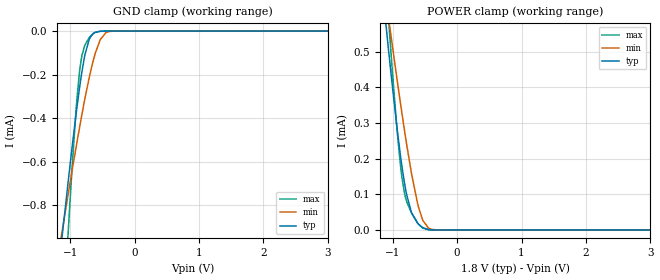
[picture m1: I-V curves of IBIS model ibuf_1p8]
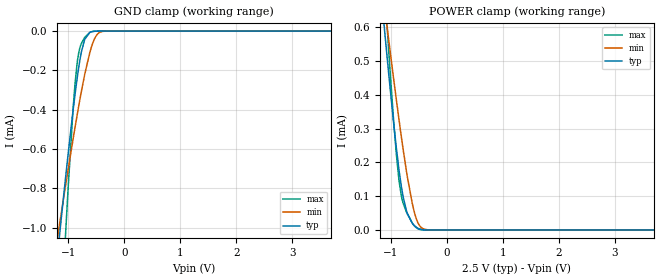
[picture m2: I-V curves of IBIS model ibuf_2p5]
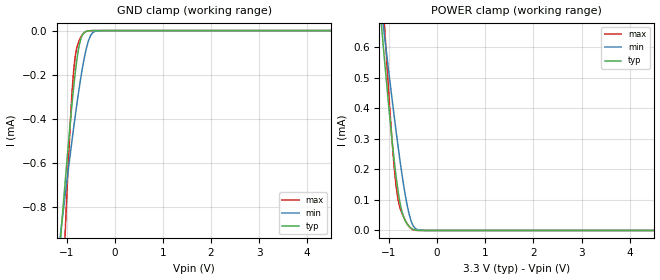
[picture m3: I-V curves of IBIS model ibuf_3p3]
|Texas Instruments Incorporated
|ISO7041 Ultra-Low Power Four-Channel Digital Isolator
[IBIS Ver]   4.1
[File name]   iso7041.ibs
[Date]   12/18/2018
[File Rev]   1.0
[Source]
| Texas Instruments Incorporated.
| Analog-eLab Design Center, HPA
| 12500 TI Blvd
| Dallas, TX -75243
[Notes]   Revision History:
| Rev 1.0: 12/18/2018
| - Initial version of the model
| - Model generated from simulations in SPECTRE
| - Warnings regarding combined Non-monotonicity of various models
|   have been reviewed and considered minor and can be ignored.
| - Model names with a trailing _1p8 contain the model for 1.8V operation.
|   Model names with a trailing _2p5 contain the model for 2.5 operation.
|   Model names with a trailing _3p3 contain the model for 3.3V operation.
|   Model names with a trailing _5p0 contain the model for 5.0V operation.
| - C_comp although listed in numerical order of value are
|   obtained from varying PVT conditions. For PVT conditions for
|   each specific value refer the buffer description under
|   respective [Model]. IBIS model user is responsible for using
|   appropriate C_comp to simulate for Signal Integrity.
[Disclaimer]
| This model is designed as an aid for customers of Texas Instruments.
| TI and its licensors and suppliers make no warranties, either expressed
| or implied, with respect to this  model, including the warranties of
| merchantability or fitness for a particular purpose. The model is
| provided solely on an "as is" basis. The entire risk as to its quality
| and performance is with the customer.
| This model is subject to change without notice. Texas Instruments
| Incorporated is not responsible for updating this model.
[Copyright]
(C) Copyright 2018 Texas Instruments Incorporated.All rights reserved.
|  Component ISO7041DBQ 16-pin QSOP - DBQ package
|  Part # ISO7041DBQ
[Component]   ISO7041DBQ
[Manufacturer]  TI
[Package]   |16 QSOP - DBQ package
|   typ   min   max
R_pkg   0.05   0.04   0.06
L_pkg   1.0nH   0.8nH   1.2nH
C_pkg   0.2pF   0.16pF   0.24pF
[Pin]  signal_name  model_name   R_pin   L_pin   C_pin
1   VCC1   power   NA   NA   NA
2   GND1   gnd   NA   NA   NA
3   INA   ibuf   NA   NA   NA
4   INB   ibuf   NA   NA   NA
5   INC   ibuf   NA   NA   NA
6   OUTD   obuf   NA   NA   NA
7   EN1   ibuf   NA   NA   NA
8   GND1   gnd   NA   NA   NA
9   GND2   gnd   NA   NA   NA
10   EN2   ibuf   NA   NA   NA
11   IND   ibuf   NA   NA   NA
12   OUTC   obuf   NA   NA   NA
13   OUTB   obuf   NA   NA   NA
14   OUTA   obuf   NA   NA   NA
15   GND2   gnd   NA   NA   NA
16   VCC2   power   NA   NA   NA
|   Model Selectors
[Model Selector] ibuf
ibuf_1p8   1.8V   digital Input
ibuf_2p5   2.5V   digital Input
ibuf_3p3   3.3V   digital Input
ibuf_5p0   5.0V   digital Input
[Model Selector] obuf
obuf_1p8   1.8V   digital Output
obuf_2p5   2.5V   digital Output
obuf_3p3   3.3V   digital Output
obuf_5p0   5.0V   digital Output
| Models and submodels in the file (8): ibuf_1p8 (Input), ibuf_2p5 (Input), ibuf_3p3 (Input), ibuf_5p0 (Input), obuf_1p8 (3-state), obuf_2p5 (3-state), obuf_3p3 (3-state), obuf_5p0 (3-state)
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|   ibuf_1p8 Model
[Model]   ibuf_1p8
Model_type   Input
Vinl = 0.54
Vinh = 1.26
|   typ   min   max
C_comp   0.001pF   0.001pF   0.017pF
[Model spec]
|subparameter
Vinl   0.54   0.513   0.567
Vinh   1.26   1.197   1.323
| Where Nom  PVT is Nominal Process, 1.8V, 27C
|   Fast PVT is Strong Process,  1.89V, -55C
|   Slow PVT is Weak Process,   1.71V, 150C
[Voltage Range]   1.8   1.71   1.89
|Junction Temperature
[Temperature Range]   27   150   -55
[Power Clamp Reference]   1.8   1.71   1.89
[GND Clamp Reference]   0   0   0
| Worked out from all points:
|   GND clamp passes 1 mA (typ) near -1.14 V on its own axis
|   POWER clamp passes 1 mA (typ) near -1.34 V on its own axis
[GND Clamp]
|   Voltage   I(typ)   I(min)   I(max)
-1.8V     -2.874mA   -2.194mA   -5.358mA
-1.163V   -1.051mA   -990.5uA   -1.631mA
-1.028V   -685.8uA   -745.5uA   -916.4uA
-963mV    -518.7uA   -630.7uA   -600.9uA
-909mV    -386.3uA   -537.1uA   -368uA
-844.2mV  -241.6uA   -428.2uA   -164.1uA
-779.4mV  -123.6uA   -324.7uA   -71.73uA
-703.8mV  -38.73uA   -214.4uA   -30.27uA
-612mV    -6.04uA    -104.4uA   -6.199uA
-531mV    -954.3nA   -38.74uA   -826.6nA
-363.6mV  -5.494nA   -1.017uA   0A
3.6V      0A         0A         0A
[POWER Clamp]
|   Voltage   I(typ)   I(min)   I(max)
-1.8V     1.872mA    1.618mA    2.859mA
-1.179V   709.7uA    751.5uA    913uA
-1.06V    499.3uA    591.4uA    584.6uA
-1.006V   407.3uA    520uA      450.5uA
-936mV    293.7uA    428.7uA    291.6uA
-882mV    214.1uA    360.3uA    188.5uA
-817.2mV  133.7uA    281.1uA    105uA
-703.8mV  47.68uA    155.5uA    46.84uA
-612mV    18.95uA    74.29uA    19.16uA
-531mV    6.472uA    26.79uA    4.999uA
-309.6mV  28.26nA    305.5nA    1.511nA
3.6V      0A         0A         0A
|   ibuf_2p5 Model
[Model]   ibuf_2p5
Model_type   Input
Vinl = 0.75
Vinh = 1.75
|   typ   min   max
C_comp   0.001pF   0.001pF   0.018pF
[Model spec]
|subparameter
Vinl   0.75   0.675   0.825
Vinh   1.75   1.575   1.925
| Where Nom  PVT is Nominal Process, 2.5V, 27C
|   Fast PVT is Strong Process,  2.75V, -55C
|   Slow PVT is Weak Process,   2.25V, 150C
[Voltage Range]   2.5   2.25   2.75
|Junction Temperature
[Temperature Range]   27   150   -55
[Power Clamp Reference]   2.5   2.25   2.75
[GND Clamp Reference]   0   0   0
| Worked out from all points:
|   GND clamp passes 1 mA (typ) near -1.14 V on its own axis
[GND Clamp]
|   Voltage   I(typ)   I(min)   I(max)
-2.5V     -4.931mA   -3.55mA    -9.6mA
-1.225V   -1.223mA   -1.105mA   -1.976mA
-1.12V    -933.2uA   -912.1uA   -1.399mA
-1.038V   -711.4uA   -762.9uA   -965.7uA
-917.5mV  -406.6uA   -551.7uA   -401.9uA
-835mV    -222.8uA   -413.1uA   -144.5uA
-782.5mV  -128.4uA   -329.5uA   -74.26uA
-707.5mV  -41.42uA   -219.5uA   -31.76uA
-617.5mV  -6.799uA   -110.1uA   -6.973uA
-497.5mV  -415.7nA   -22.1uA    -306.4nA
-355mV    -1.124nA   -814.4nA   0A
5V        0A         0A         0A
[POWER Clamp]
|   Voltage   I(typ)   I(min)   I(max)
-2.5V     3.216mA    2.616mA    5.124mA
-1.113V   590.9uA    661.5uA    723.9uA
-1.083V   538.1uA    621.2uA    642.9uA
-1.03V    447.4uA    551.3uA    508.4uA
-902.5mV  243.2uA    386.1uA    224.8uA
-857.5mV  181.3uA    329.9uA    151uA
-812.5mV  128.7uA    275.6uA    100.9uA
-707.5mV  49.45uA    159.3uA    48.16uA
-602.5mV  17.04uA    67.35uA    16.93uA
-512.5mV  4.733uA    19.94uA    3.316uA
-287.5mV  10.54nA    180.4nA    0A
5V        0A         0A         0A
|   ibuf_3p3 Model
[Model]   ibuf_3p3
Model_type   Input
Vinl = 0.99
Vinh = 2.31
|   typ   min   max
C_comp   0.001pF   0.001pF   0.019pF
[Model spec]
|subparameter
Vinl   0.99   0.9   1.08
Vinh   2.31   2.1   2.52
| Where Nom  PVT is Nominal Process, 3.3V, 27C
|   Fast PVT is Strong Process,  3.6V, -55C
|   Slow PVT is Weak Process,   3.0V, 150C
[Voltage Range]   3.3   3   3.6
|Junction Temperature
[Temperature Range]   27   150   -55
[Power Clamp Reference]   3.3   3   3.6
[GND Clamp Reference]   0   0   0
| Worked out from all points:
|   GND clamp passes 1 mA (typ) near -1.14 V on its own axis
|   POWER clamp passes 1 mA (typ) near -1.34 V on its own axis
[GND Clamp]
|   Voltage   I(typ)   I(min)   I(max)
-3.3V     -7.303mA   -5.115mA   -14.49mA
-1.112V   -911.7uA   -897.7uA   -1.357mA
-1.033V   -699.3uA   -754.6uA   -942.3uA
-1.023V   -673.2uA   -736.9uA   -892.2uA
-904.2mV  -375uA     -528.9uA   -349.4uA
-844.8mV  -242.8uA   -429.2uA   -165.4uA
-795.3mV  -149.2uA   -349.4uA   -86.15uA
-735.9mV  -67.03uA   -259.5uA   -44.63uA
-597.3mV  -4.377uA   -89.99uA   -4.461uA
-458.7mV  -146.1nA   -10.13uA   -80.81nA
-260.7mV  -4.623nA   -64.29nA   0A
6.6V      0A         0A         0A
[POWER Clamp]
|   Voltage   I(typ)   I(min)   I(max)
-3.3V     4.765mA    3.768mA    7.732mA
-1.171V   696.2uA    741.3uA    891.2uA
-1.132V   625.3uA    687.6uA    777.9uA
-1.092V   555.3uA    634.3uA    669uA
-943.8mV  305.9uA    438.7uA    308.2uA
-854.7mV  177.7uA    326.5uA    147.2uA
-785.4mV  102.5uA    243.9uA    81.85uA
-706.2mV  48.82uA    157.9uA    47.7uA
-597.3mV  16.05uA    63.69uA    15.77uA
-508.2mV  4.382uA    18.55uA    2.996uA
-260.7mV  116.9nA    91.25nA    0A
6.6V      0A         0A         0A
